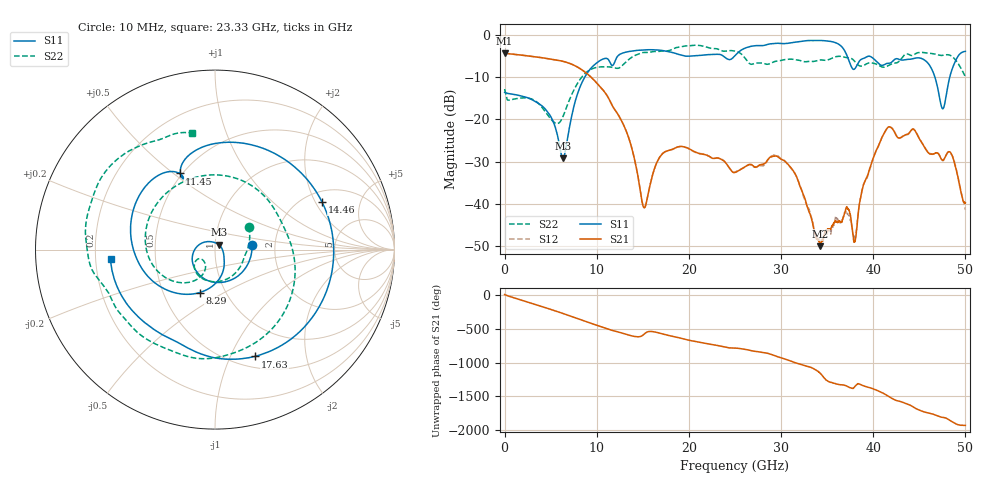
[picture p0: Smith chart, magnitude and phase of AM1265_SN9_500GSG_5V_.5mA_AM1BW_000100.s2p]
!Keysight Technologies,N5245B,MY58422270,A.16.20.02
!Date: Thursday, March 05, 2026 00:28:26
!Correction: S11(C  2-Port  )
!S21(C  2-Port  )
!S12(C  2-Port  )
!S22(C  2-Port  )
!S2P File: Measurements: S11, S21, S12, S22:
# Hz S  dB  R 50
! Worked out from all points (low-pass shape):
!   3201 points, 10 MHz to 50 GHz, reference 50 ohm
!   highest |S21| = -4.41 dB at 10 MHz (marker M1); lowest = -50.0 dB at 34.25 GHz (marker M2)
!   |S21| within 3 dB of the highest: start of sweep to 7.697 GHz
!   lowest |S11| = -29.2 dB at 6.337 GHz (marker M3), VSWR 1.07, Z = 52.1 + j2.83 ohm
!   |S11| at or under -10 dB: start of sweep to 8.721 GHz; 46.69 GHz to 48.31 GHz (1.623 GHz wide, 3.42 % of centre)
!   |S22| runs from -21.0 to -2.5 dB; largest |S21 - S12| = 0.0098
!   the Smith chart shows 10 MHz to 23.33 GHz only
!   S11 on the Smith chart (normalised r, x): 10 MHz: 1.52, +0.08; 8.29 GHz: 0.76, -0.39; 11.45 GHz: 0.48, +0.53; 14.46 GHz: 2.45, +2.27; 17.63 GHz: 0.62, -1.24; 23.33 GHz: 0.26, -0.04
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1e7  -13.66 6.7  -4.41 4.2  -4.52 3.6  -12.87 34.0
1.931491e9  -14.57 -77.3  -4.87 -82.7  -4.87 -82.7  -14.95 -86.0
3.852981e9  -16.50 -143.5  -5.40 -164.5  -5.40 -164.4  -16.65 -141.7
6.336859e9  -29.22 51.5  -6.31 84.8  -6.32 84.9  -19.41 -119.4
8.289594e9  -11.88 -109.8  -8.17 -8.5  -8.16 -8.4  -10.31 -146.9
8.352081e9  -11.57 -112.6  -8.26 -11.5  -8.25 -11.4  -10.13 -148.8
1.144521e10  -6.59 115.0  -15.72 -156.3  -15.72 -156.2  -7.65 74.9
1.446023e10  -3.71 24.1  -33.28 100.6  -33.27 101.0  -4.65 -79.8
1.521008e10  -3.59 0.1  -40.89 147.5  -40.79 147.5  -4.23 -106.3
1.667854e10  -3.64 -43.8  -29.53 159.4  -29.57 159.6  -3.98 -141.2
1.763148e10  -3.95 -69.6  -27.50 125.4  -27.48 125.7  -3.87 -157.9
2.333346e10  -4.68 -174.7  -29.29 -35.3  -29.31 -35.2  -3.59 101.3
2.5005e10  -4.97 173.6  -32.60 -66.5  -32.44 -66.7  -3.90 70.8
2.95041e10  -2.05 95.8  -28.69 172.6  -28.50 171.7  -6.27 -19.4
3.334708e10  -1.39 35.6  -43.76 1.5  -43.57 -0.1  -6.34 -127.7
3.425315e10  -1.38 19.9  -50.01 -79.2  -48.52 -91.7  -5.99 -146.7
3.670578e10  -3.17 -31.6  -43.42 110.9  -43.37 107.0  -5.23 165.0
3.801802e10  -8.04 -25.9  -48.91 86.8  -47.86 94.0  -6.40 139.1
4.167354e10  -6.78 -54.2  -21.82 -59.6  -21.79 -60.0  -7.28 116.3
4.511035e10  -5.55 -102.4  -24.97 91.2  -24.95 91.3  -4.20 75.8
4.770358e10  -16.85 69.9  -29.36 -13.3  -29.47 -13.0  -4.83 40.0
5e10  -3.95 -73.2  -39.76 -129.0  -41.44 -119.8  -9.85 2.6
